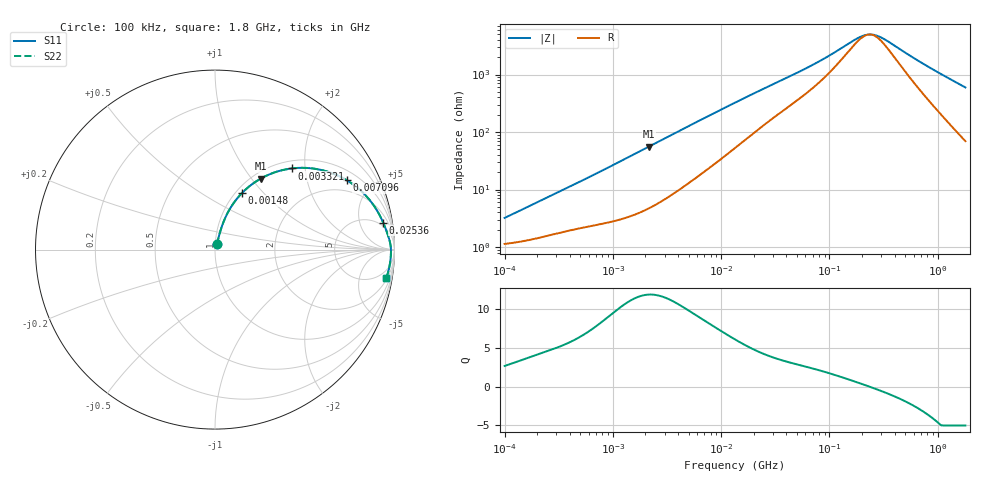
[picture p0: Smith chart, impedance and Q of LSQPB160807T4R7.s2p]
! LSQPB160807T4R7  S-PARAMETER MODEL  ( General Type )
! Model Generated by TAIYO YUDEN Corporation (http://www.ty-top.com)
! Version 1.0
! TAIYO YUDEN Control No. 110308NG25SB-FKC
! Copyright(c) 2011 TAIYO YUDEN CO.,LTD. All Rights Reserved.
! Product Description (link to TY-COMPAS)
! https://ds.yuden.co.jp/TYCOMPAS/or/detail?pn=LSQPB160807T4R7M&u=M
! Products Name : Inductors
! Characteristics :
!  Inductance : 4.7 uH , SRF(min) : 150 MHz , DC Resistance(max) : 1.3 Ohm
!  Rated Current : Saturation :240 mA , Temp Rise : 310 mA (40 degC)
!  Case Size : 1.6 x 0.8 / 0.063 x 0.031 [mm/inch] , Thickness : 0.7 / 0.028 [mm/inch]
!  (Conditions: Temperature = 25 degC , DC Bias Current/Voltage = 0A / 0V)
! External Node Assignments :
!  1  o---GGG---o  2
! GND o---------o GND
! Frequency Range : 0.1MHz  -  1800MHz  [ 402 STEP ]
# MHz S RI R 50
! Freq[MHz].  S11 Real  S11 Imag  S21 Real  S21 Imag  S12 Real  S12 Imag  S22 Real  S22 Imag
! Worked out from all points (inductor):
!   401 points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, 100 kHz to 1.8 GHz, reference 50 ohm
!   read as one part in series: L = 4.72 uH near 118.7 kHz
!   highest Q = 11.8 at 2.137 MHz (marker M1), where L = 4.13 uH
!   self-resonance near 233.3 MHz
!   S11 on the Smith chart (normalised r, x): 100 kHz: 1.02, +0.06; 1.48 MHz: 1.07, +0.77; 3.321 MHz: 1.15, +1.70; 7.096 MHz: 1.42, +3.52; 25.36 MHz: 4, +11; 1.8 GHz: 2, -12
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0.1  0.0121 0.0294  0.9879 -0.0294  0.9879 -0.0294  0.0121 0.0294
0.247521  0.0202 0.0687  0.9798 -0.0687  0.9798 -0.0687  0.0202 0.0687
0.516129  0.0393 0.1322  0.9607 -0.1322  0.9607 -0.1322  0.0393 0.1322
0.929126  0.0791 0.2205  0.9209 -0.2205  0.9209 -0.2205  0.0791 0.2205
1.479789  0.152 0.3169  0.848 -0.3169  0.848 -0.3169  0.152 0.3169
2.136843  0.2538 0.395  0.7462 -0.395  0.7462 -0.395  0.2538 0.395
2.66389  0.3354 0.4313  0.6646 -0.4313  0.6646 -0.4313  0.3354 0.4313
3.320932  0.4283 0.4522  0.5717 -0.4522  0.5717 -0.4522  0.4283 0.4522
4.679446  0.5785 0.4465  0.4215 -0.4465  0.4215 -0.4465  0.5785 0.4465
7.096489  0.7349 0.3861  0.2651 -0.3861  0.2651 -0.3861  0.7349 0.3861
9.75753  0.8207 0.3206  0.1793 -0.3206  0.1793 -0.3206  0.8207 0.3206
13.41641  0.8782 0.2548  0.1218 -0.2548  0.1218 -0.2548  0.8782 0.2548
25.36465  0.9369 0.1507  0.0631 -0.1507  0.0631 -0.1507  0.9369 0.1507
69.24595  0.9701 0.0597  0.0299 -0.0597  0.0299 -0.0597  0.9701 0.0597
102.472  0.9757 0.0372  0.0243 -0.0372  0.0243 -0.0372  0.9757 0.0372
171.3985  0.9794 0.013  0.0206 -0.013  0.0206 -0.013  0.9794 0.013
208.5031  0.98 0.00471  0.02 -0.00471  0.02 -0.00471  0.98 0.00471
235.6695  0.9803 -0.000424  0.0197 0.000424  0.0197 0.000424  0.9803 -0.000424
266.3756  0.9804 -0.00558  0.0196 0.00558  0.0196 0.00558  0.9804 -0.00558
357.3983  0.9804 -0.0185  0.0196 0.0185  0.0196 0.0185  0.9804 -0.0185
782.6622  0.9768 -0.0643  0.0232 0.0643  0.0232 0.0643  0.9768 -0.0643
1800  0.9553 -0.1562  0.0447 0.1562  0.0447 0.1562  0.9553 -0.1562
